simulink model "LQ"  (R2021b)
settings: Solver=VariableStepAuto  StartTime=0.0  StopTime=5  RelTol=1e-3
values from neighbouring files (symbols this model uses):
  a = 0.27    [CompareGazeboSimulink.m]    (also in RobotModel.m)
  b = 0.31    [CompareGazeboSimulink.m]    (also in RobotModel.m)
  desired_ang = 1    [RobotModel.m]
  desired_vel = 2    [RobotModel.m]
  distAng = 0    [RobotModel.m]
  distVel = 0    [RobotModel.m]
  fro = 0.02    [CompareGazeboSimulink.m]    (also in RobotModel.m)
  fsl = 0.8    [CompareGazeboSimulink.m]    (also in RobotModel.m)
  fsly = 0.8    [CompareGazeboSimulink.m]    (also in RobotModel.m)
  I = (1/12)*m*((2*t)^2 + 0.12^2) + 1.5    (= 2.384)    [CompareGazeboSimulink.m]    (also in RobotModel.m = 0.866666666667)
  k = 1    [RobotModel.m]
  ko = 0    [CompareGazeboSimulink.m]    (also in RobotModel.m = 0.25)
  kt = 0.58    [CompareGazeboSimulink.m]    (also in RobotModel.m)
  m = 51    [CompareGazeboSimulink.m]    (also in RobotModel.m = 50)
  mdy = 10    [CompareGazeboSimulink.m]    (also in RobotModel.m)
  mst = 10    [CompareGazeboSimulink.m]    (also in RobotModel.m)
  Q = [1 0    [RobotModel.m]
  r = 0.19    [CompareGazeboSimulink.m]    (also in RobotModel.m)
  R = [0.01 0    [RobotModel.m]
  T_vel_variance = 0.0005    [RobotModel.m]
  Th0 = 0    [CompareGazeboSimulink.m]    (also in RobotModel.m = 0.9714)
  Th_vel0 = 0    [CompareGazeboSimulink.m]    (also in RobotModel.m)
  Ts = 0.01    [CompareGazeboSimulink.m]    (also in RobotModel.m = 0.05)
  X0 = 0    [CompareGazeboSimulink.m]    (also in RobotModel.m)
  x_vel0 = 0    [CompareGazeboSimulink.m]    (also in RobotModel.m)
  x_vel_variance = 0.0005    [RobotModel.m]
  Y0 = 0    [CompareGazeboSimulink.m]    (also in RobotModel.m = 2.5)
libraries: mobileRoboticsLib x1

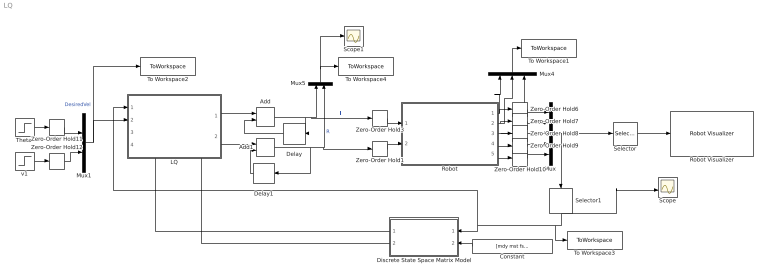
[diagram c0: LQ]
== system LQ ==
  Add : Sum
  Add1 : Sum
  Constant : Constant  Value=[mdy mst fsly r t a b m I Ts k]
  Delay : Delay  DelayLength=1
  Delay1 : Delay  DelayLength=1
  Discrete State Space Matrix Model : MATLAB Function  TreatAsAtomicUnit=on
  LQ : Subsystem
  Mux : Mux  Inputs=5
  Mux1 : Mux  Inputs=2
  Mux4 : Mux  Inputs=3
  Mux5 : Mux  Inputs=2
  Robot : Subsystem
  Robot Visualizer : mobileRoboticsLib/Environments/Robot Visualizer  robotRadius=0.3  showTrajectory=on  hasWaypoints=off  hasLidar=off  sensorOffset=[ 0, 0 ]  scanAngles=[ -pi/4, 0, pi/4 ]  hasObjDetector=off  objDetectorOffset=[ 0, 0 ]  objDetectorAngle=0  objDetectorFOV=pi/4  objDetectorMaxRange=5  objectColors=[ 1, 0, 0; 0, 1, 0; 0, 0, 1 ]  objectMarkers=s
  Scope : Scope  NumInputPorts=2
  Scope1 : Scope
  Selector : Selector  InputPortWidth=5  IndexOptions=Index vector (dialog)  Indices=[1 2 3]  OutputSizes=1
  Selector1 : Selector  InputPortWidth=5  IndexOptions=Index vector (dialog)  Indices=[4 5]  OutputSizes=1
  Theta' : Step  After=desired_ang  SampleTime=0
  To Workspace1 : ToWorkspace  VariableName=ActualPos  SaveFormat=Timeseries  SampleTime=-1
  To Workspace2 : ToWorkspace  VariableName=DesiredVel  SaveFormat=Timeseries  SampleTime=-1
  To Workspace3 : ToWorkspace  VariableName=ActualVel  SaveFormat=Timeseries  SampleTime=-1
  To Workspace4 : ToWorkspace  VariableName=Forces  SaveFormat=Timeseries  SampleTime=-1
  Zero-Order Hold{1,3,6..12} (9 alike) : ZeroOrderHold  SampleTime=Ts
  v1 : Step  After=desired_vel  SampleTime=0
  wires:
  Zero-Order Hold12/1 -> Mux1/2
  Zero-Order Hold11/1 -> Mux1/1
  Theta'/1 -> Zero-Order Hold11/1
  v1/1 -> Zero-Order Hold12/1
  Mux4/1 -> To Workspace1/1
  Selector1/1 -> Scope/2, To Workspace3/1, LQ/1(Actual State), Discrete State Space Matrix Model/1(State)
  Discrete State Space Matrix Model/1(A) -> LQ/3(A)
  Robot/5(v) -> Zero-Order Hold10/1
  Robot/4(Theta') -> Zero-Order Hold9/1
  Selector/1 -> Robot Visualizer/1
  Mux1/1 -> To Workspace2/1, LQ/2(Desired State)  "DesiredVel"
  Zero-Order Hold7/1 -> Mux/2
  Robot/2(Y) -> Mux4/2, Zero-Order Hold7/1
  Delay/1 -> Add/2
  Zero-Order Hold10/1 -> Mux/5
  Robot/1(X) -> Mux4/1, Zero-Order Hold6/1
  Zero-Order Hold1/1 -> Robot/2(Right Force)
  Zero-Order Hold6/1 -> Mux/1
  Zero-Order Hold8/1 -> Mux/3
  Delay1/1 -> Add1/2
  Add/1 -> Mux5/1, Zero-Order Hold3/1, Delay/1  "L"
  Zero-Order Hold9/1 -> Mux/4
  Discrete State Space Matrix Model/2(B) -> LQ/4(B)
  Robot/3(Theta) -> Mux4/3, Zero-Order Hold8/1
  LQ/2(Right Force) -> Add1/1
  Zero-Order Hold3/1 -> Robot/1(Left Force)
  LQ/1(" Left Force") -> Add/1
  Mux/1 -> Selector/1, Selector1/1
  Constant/1 -> Discrete State Space Matrix Model/2(param)
  Add1/1 -> Zero-Order Hold1/1, Mux5/2, Delay1/1  "R"
  Mux5/1 -> To Workspace4/1, Scope1/1

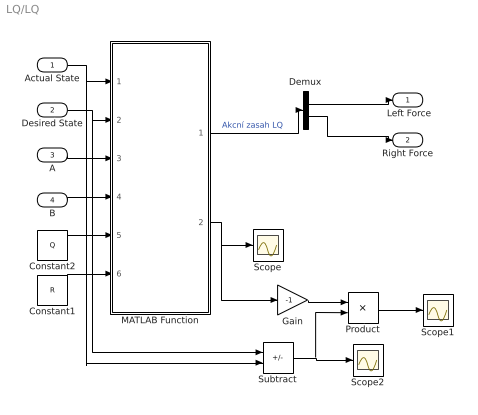
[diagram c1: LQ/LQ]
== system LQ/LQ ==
  Actual State : Inport
  Desired State : Inport  Port=2
  A : Inport  Port=3
  B : Inport  Port=4
  Constant1 : Constant  Value=R
  Constant2 : Constant  Value=Q
  Demux : Demux  Outputs=2
  Gain : Gain  Gain=-1
  MATLAB Function : MATLAB Function  TreatAsAtomicUnit=on
  Product : Product  Multiplication=Matrix(*)
  Scope : Scope
  Scope1 : Scope
  Scope2 : Scope
  Subtract : Sum  Inputs=+-
  " Left Force" : Outport
  Right Force : Outport  Port=2
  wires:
  MATLAB Function/1(u) -> Demux/1  "Akcní zasah LQ"
  Actual State/1 -> Subtract/2, MATLAB Function/1(ActualState)
  Desired State/1 -> Subtract/1, MATLAB Function/2(DesiredState)
  A/1 -> MATLAB Function/3(A)
  B/1 -> MATLAB Function/4(B)
  Constant2/1 -> MATLAB Function/5(Q)
  Constant1/1 -> MATLAB Function/6(R)
  MATLAB Function/2(K) -> Gain/1, Scope/1
  Subtract/1 -> Scope2/1, Product/2
  Gain/1 -> Product/1
  Product/1 -> Scope1/1
  Demux/1 -> " Left Force"/1
  Demux/2 -> Right Force/1

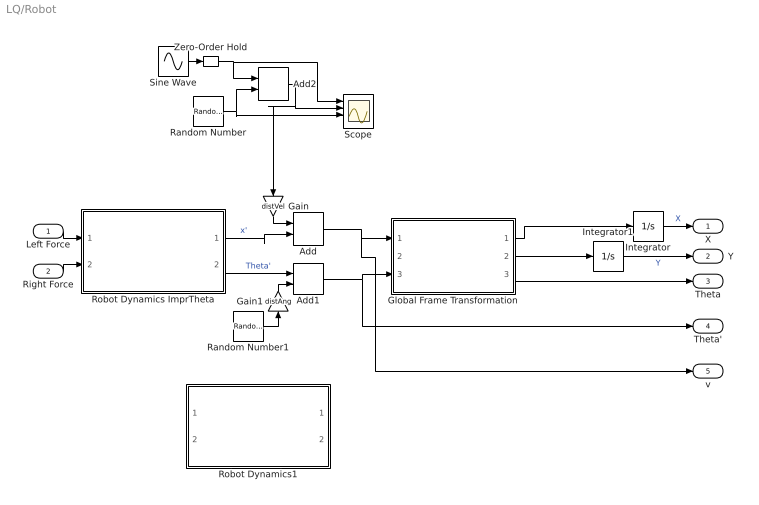
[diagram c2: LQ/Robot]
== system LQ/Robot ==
  Left Force : Inport
  Right Force : Inport  Port=2
  Add : Sum
  Add1 : Sum
  Add2 : Sum
  Gain : Gain  Gain=distVel
  Gain1 : Gain  Gain=distAng
  Global Frame Transformation : Subsystem
  Integrator : Integrator  InitialCondition=X0
  Integrator1 : Integrator  InitialCondition=Y0
  Random Number : RandomNumber  Variance=x_vel_variance  SampleTime=0.2
  Random Number1 : RandomNumber  Variance=T_vel_variance  SampleTime=0.2
  Robot Dynamics ImprTheta : Subsystem
  Robot Dynamics1 : Subsystem  Commented=on
  Scope : Scope  NumInputPorts=4
  Sine Wave : Sin  Amplitude=0.1*desired_vel  Frequency=0.2  SampleTime=0
  Zero-Order Hold : ZeroOrderHold  SampleTime=0.25
  X : Outport
  Y : Outport  Port=2
  Theta : Outport  Port=3
  Theta' : Outport  Port=4
  v : Outport  Port=5
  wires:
  Right Force/1 -> Robot Dynamics ImprTheta/2(Right Force)
  Global Frame Transformation/1(X') -> Integrator/1
  Integrator/1 -> X/1  "X"
  Left Force/1 -> Robot Dynamics ImprTheta/1(Left Force)
  Global Frame Transformation/2(Y') -> Integrator1/1
  Global Frame Transformation/3(Theta) -> Theta/1
  Integrator1/1 -> Y/1  "Y"
  Robot Dynamics ImprTheta/1(x') -> Add/2  "x'"
  Add/1 -> v/1, Global Frame Transformation/1(x')
  Robot Dynamics ImprTheta/2(Theta') -> Add1/1  "Theta'"
  Add1/1 -> Theta'/1, Global Frame Transformation/3(Theta')
  Random Number1/1 -> Gain1/1
  Random Number/1 -> Add2/2, Scope/3
  Add2/1 -> Gain/1, Scope/2
  Sine Wave/1 -> Zero-Order Hold/1
  Zero-Order Hold/1 -> Scope/1, Add2/1
  Gain/1 -> Add/1
  Gain1/1 -> Add1/2

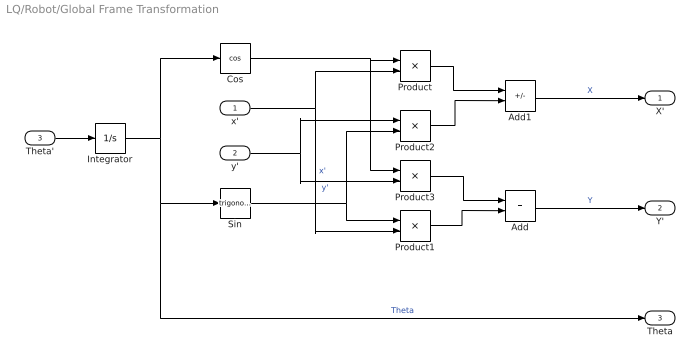
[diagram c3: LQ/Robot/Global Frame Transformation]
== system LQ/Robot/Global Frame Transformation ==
  x' : Inport
  y' : Inport  Port=2
  Theta' : Inport  Port=3
  Add : Sum
  Add1 : Sum  Inputs=+-
  Cos : Trigonometry  Operator=cos
  Integrator : Integrator  InitialCondition=Th0
  Product{,1..3} (4 alike) : Product
  Sin : Trigonometry
  X' : Outport
  Y' : Outport  Port=2
  Theta : Outport  Port=3
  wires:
  Add/1 -> Y'/1  "Y"
  Integrator/1 -> Theta/1, Sin/1, Cos/1  "Theta"
  Product1/1 -> Add/2
  x'/1 -> Product/2, Product1/2  "x'"
  Sin/1 -> Product1/1, Product2/2
  Product2/1 -> Add1/2
  Product3/1 -> Add/1
  Product/1 -> Add1/1
  Cos/1 -> Product/1, Product3/1
  y'/1 -> Product3/2, Product2/1  "y'"
  Add1/1 -> X'/1  "X"
  Theta'/1 -> Integrator/1

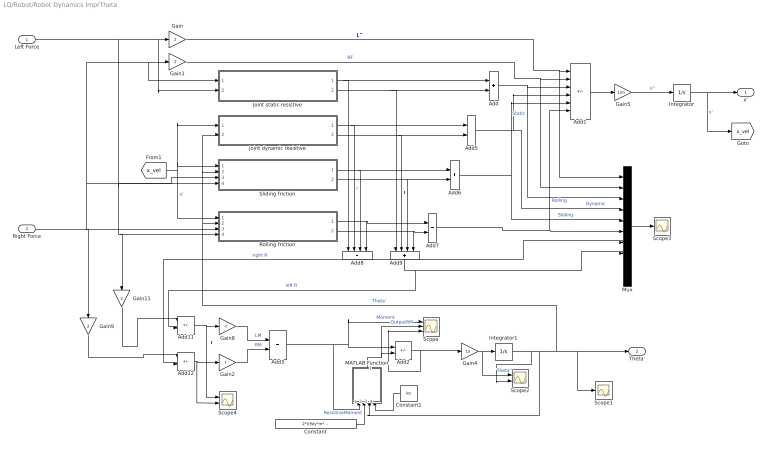
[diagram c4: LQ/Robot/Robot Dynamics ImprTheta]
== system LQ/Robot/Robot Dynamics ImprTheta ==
  Left Force : Inport
  Right Force : Inport  Port=2
  Add{,3,5..7} (5 alike) : Sum
  Add1 : Sum  Inputs=++----
  Add11 : Sum  Inputs=+-
  Add12 : Sum  Inputs=+-
  Add2 : Sum  Inputs=+-
  Add8 : Sum  Inputs=++++
  Add9 : Sum  Inputs=++++
  Constant : Constant  Value=2*((fsly*m*9.81)/(a+b))*a*b*kt
  Constant1 : Constant  Value=ko
  Gain{,1,9,11} (4 alike) : Gain  Gain=2
  Gain2 : Gain  Gain=t
  Gain4 : Gain  Gain=1/I
  Gain5 : Gain  Gain=1/m
  Gain8 : Gain  Gain=-t
  Integrator : Integrator  InitialCondition=x_vel0
  Integrator1 : Integrator  InitialCondition=Th_vel0
  Joint dynamic resistive : Subsystem
  Joint static resistive : Subsystem
  MATLAB Function : MATLAB Function  TreatAsAtomicUnit=on
  Mux : Mux  Inputs=10
  Rolling friction : Subsystem
  Scope : Scope  NumInputPorts=3
  Scope1 : Scope
  Scope2 : Scope  NumInputPorts=2
  Scope3 : Scope
  Scope4 : Scope  NumInputPorts=2
  Sliding friction : Subsystem
  x' : Outport
  Theta' : Outport  Port=2
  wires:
  Gain4/1 -> Scope2/1, Integrator1/1  "Theta''"
  Integrator1/1 -> Scope2/2, Sliding friction/2(Theta'), Joint dynamic resistive/2(Theta'), Rolling friction/2(Theta'), Scope1/1, Theta'/1, MATLAB Function/3(Omega)  "Theta'"
  Gain1/1 -> Mux/2, Add1/2  "RF"
  Add1/1 -> Gain5/1
  Gain5/1 -> Integrator/1  "x''"
  Integrator/1 -> x'/1, [x_vel]  "x'"
  [x_vel] -> Joint dynamic resistive/1("Local Long Velocity "), Sliding friction/1(Local longitudal velocity), Rolling friction/1(Local longitudal velocity)  "x'"
  Joint static resistive/2(Static Resistive Force Left) -> Add9/1, Add/2
  Joint dynamic resistive/1(Dynamic Resistive Force Right) -> Add8/2, Add5/1  "r"
  Joint dynamic resistive/2(Dynamic Resistive Force Left) -> Add9/2, Add5/2  "l"
  Sliding friction/1(Friction Right Force) -> Add8/3, Add6/1
  Sliding friction/2(Friction Left Force) -> Add9/3, Add6/2
  Rolling friction/1(Friction Right Force) -> Add8/4, Add7/1
  Rolling friction/2(Friction Left Force) -> Add9/4, Add7/2
  Add/1 -> Add1/3, Mux/3  "Static"
  Add6/1 -> Add1/5, Mux/5  "Sliding"
  Add7/1 -> Mux/6, Add1/6  "Rolling"
  Add5/1 -> Mux/4, Add1/4  "Dynamic"
  Add9/1 -> Add11/2, Mux/8  "left R"
  Add8/1 -> Add12/2, Mux/7  "right R"
  Mux/1 -> Scope3/1
  Add11/1 -> Scope4/1, Gain8/1  "LL"
  Add12/1 -> Scope4/2, Gain2/1
  Gain9/1 -> Add12/1
  Gain11/1 -> Add11/1
  Gain8/1 -> Add3/1  "LM"
  Gain2/1 -> Add3/2  "RM"
  Gain/1 -> Mux/1, Add1/1  "LF"
  Joint static resistive/1(Static Resistive Force Right) -> Add8/1, Add/1
  Add2/1 -> Scope/3, Gain4/1
  Add3/1 -> Scope/1, Add2/1, MATLAB Function/1(Moment)  "Moment"
  MATLAB Function/1(y) -> Scope/2, Add2/2  "OutputRM"
  Constant/1 -> MATLAB Function/2(ResistiveMoment)  "ResistiveMoment"
  Left Force/1 -> Gain11/1, Rolling friction/4(Fl), Sliding friction/4(Fl), Joint static resistive/2("Fl "), Gain/1
  Right Force/1 -> Gain9/1, Rolling friction/3(Fr), Sliding friction/3(Fr), Joint static resistive/1(Fr), Gain1/1
  Constant1/1 -> MATLAB Function/4(ko)

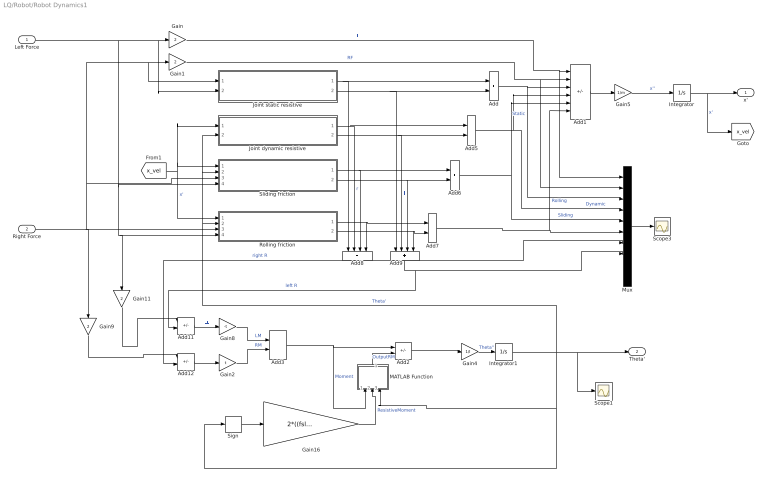
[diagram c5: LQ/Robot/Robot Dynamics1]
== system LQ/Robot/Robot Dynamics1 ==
  Left Force : Inport
  Right Force : Inport  Port=2
  Add{,3,5..7} (5 alike) : Sum
  Add1 : Sum  Inputs=++----
  Add11 : Sum  Inputs=+-
  Add12 : Sum  Inputs=+-
  Add2 : Sum  Inputs=+-
  Add8 : Sum  Inputs=++++
  Add9 : Sum  Inputs=++++
  Gain{,1,9,11} (4 alike) : Gain  Gain=2
  Gain16 : Gain  Gain=2*((fsly*m*9.81)/(a+b))*a*b
  Gain2 : Gain  Gain=t
  Gain4 : Gain  Gain=1/I
  Gain5 : Gain  Gain=1/m
  Gain8 : Gain  Gain=-t
  Integrator : Integrator  InitialCondition=x_vel0
  Integrator1 : Integrator  InitialCondition=Th_vel0
  Joint dynamic resistive : Subsystem
  Joint static resistive : Subsystem
  MATLAB Function : MATLAB Function  TreatAsAtomicUnit=on
  Mux : Mux  Inputs=10
  Rolling friction : Subsystem
  Scope1 : Scope
  Scope3 : Scope
  Sign : Signum
  Sliding friction : Subsystem
  x' : Outport
  Theta' : Outport  Port=2
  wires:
  Right Force/1 -> Rolling friction/3(Fr), Sliding friction/3(Fr), Joint static resistive/1(Fr), Gain1/1, Gain9/1
  Gain4/1 -> Integrator1/1  "Theta''"
  Integrator1/1 -> Sliding friction/2(Theta'), Joint dynamic resistive/2(Theta'), Rolling friction/2(Theta'), MATLAB Function/3(Omega), Sign/1, Scope1/1, Theta'/1  "Theta'"
  Left Force/1 -> Rolling friction/4(Fl), Gain11/1, Sliding friction/4(Fl), Joint static resistive/2("Fl "), Gain/1
  Gain1/1 -> Mux/2, Add1/2  "RF"
  Add1/1 -> Gain5/1
  Gain5/1 -> Integrator/1  "x''"
  Integrator/1 -> x'/1, [x_vel]  "x'"
  [x_vel] -> Joint dynamic resistive/1("Local Long Velocity "), Sliding friction/1(Local longitudal velocity), Rolling friction/1(Local longitudal velocity)  "x'"
  Joint static resistive/2(Static Resistive Force Left) -> Add9/1, Add/2
  Joint dynamic resistive/1(Dynamic Resistive Force Right) -> Add8/2, Add5/1  "r"
  Joint dynamic resistive/2(Dynamic Resistive Force Left) -> Add9/2, Add5/2  "l"
  Sliding friction/1(Friction Right Force) -> Add8/3, Add6/1
  Sliding friction/2(Friction Left Force) -> Add9/3, Add6/2
  Rolling friction/1(Friction Right Force) -> Add8/4, Add7/1
  Rolling friction/2(Friction Left Force) -> Add9/4, Add7/2
  Add/1 -> Add1/3, Mux/3  "Static"
  Add6/1 -> Add1/5, Mux/5  "Sliding"
  Add7/1 -> Mux/6, Add1/6  "Rolling"
  Add5/1 -> Mux/4, Add1/4  "Dynamic"
  Add9/1 -> Add11/2, Mux/8  "left R"
  Add8/1 -> Add12/2, Mux/7  "right R"
  Mux/1 -> Scope3/1
  Add11/1 -> Gain8/1  "LL"
  Add12/1 -> Gain2/1
  Gain9/1 -> Add12/1
  Gain11/1 -> Add11/1
  Gain8/1 -> Add3/1  "LM"
  Gain2/1 -> Add3/2  "RM"
  Gain/1 -> Mux/1, Add1/1  "LF"
  Joint static resistive/1(Static Resistive Force Right) -> Add8/1, Add/1
  Sign/1 -> Gain16/1
  Add2/1 -> Gain4/1
  Add3/1 -> Add2/1, MATLAB Function/1(Moment)  "Moment"
  MATLAB Function/1(y) -> Add2/2  "OutputRM"
  Gain16/1 -> MATLAB Function/2(ResistiveMoment)  "ResistiveMoment"

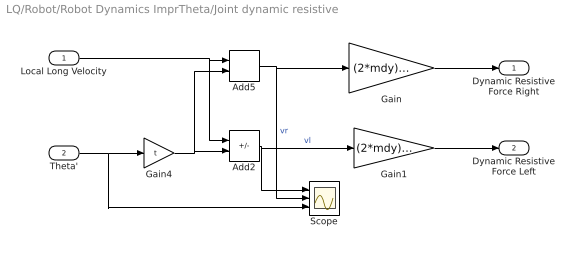
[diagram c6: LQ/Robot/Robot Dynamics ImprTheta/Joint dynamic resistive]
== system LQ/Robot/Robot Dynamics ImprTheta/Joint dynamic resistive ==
  "Local Long Velocity " : Inport
  Theta' : Inport  Port=2
  Add2 : Sum  Inputs=+-
  Add5 : Sum
  Gain : Gain  Gain=(2*mdy)/(r*r)
  Gain1 : Gain  Gain=(2*mdy)/(r*r)
  Gain4 : Gain  Gain=t
  Scope : Scope  NumInputPorts=3
  Dynamic Resistive Force Right : Outport
  Dynamic Resistive Force Left : Outport  Port=2
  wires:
  Gain/1 -> Dynamic Resistive Force Right/1
  Gain1/1 -> Dynamic Resistive Force Left/1
  Gain4/1 -> Add5/2, Add2/2
  Theta'/1 -> Scope/3, Gain4/1
  Add5/1 -> Scope/2, Gain/1  "vr"
  Add2/1 -> Scope/1, Gain1/1  "vl"
  "Local Long Velocity "/1 -> Add2/1, Add5/1

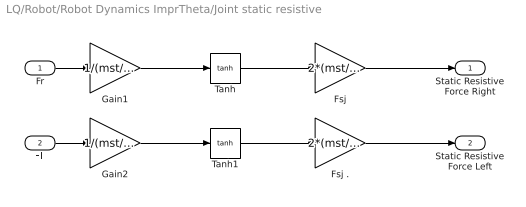
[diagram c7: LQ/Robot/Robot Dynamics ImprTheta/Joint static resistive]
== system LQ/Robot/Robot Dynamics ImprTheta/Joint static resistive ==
  Fr : Inport
  "Fl " : Inport  Port=2
  Fsj : Gain  Gain=2*(mst/r)
  Fsj . : Gain  Gain=2*(mst/r)
  Gain1 : Gain  Gain=1/(mst/r)
  Gain2 : Gain  Gain=1/(mst/r)
  Tanh : Trigonometry  Operator=tanh
  Tanh1 : Trigonometry  Operator=tanh
  Static Resistive Force Right : Outport
  Static Resistive Force Left : Outport  Port=2
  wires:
  Fr/1 -> Gain1/1
  "Fl "/1 -> Gain2/1
  Tanh/1 -> Fsj/1
  Tanh1/1 -> Fsj ./1
  Gain1/1 -> Tanh/1
  Gain2/1 -> Tanh1/1
  Fsj/1 -> Static Resistive Force Right/1
  Fsj ./1 -> Static Resistive Force Left/1

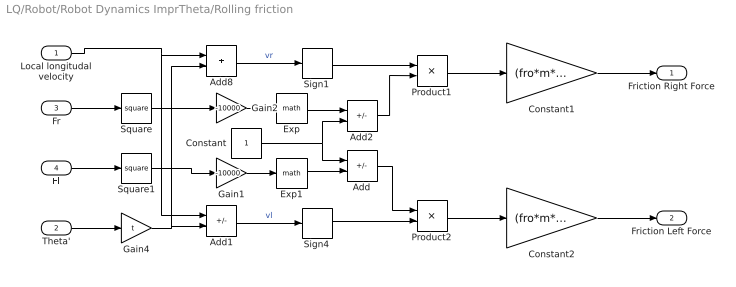
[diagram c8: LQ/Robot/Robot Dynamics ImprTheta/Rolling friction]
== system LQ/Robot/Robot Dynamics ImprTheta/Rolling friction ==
  Local longitudal velocity : Inport
  Theta' : Inport  Port=2
  Fr : Inport  Port=3
  Fl : Inport  Port=4
  Add : Sum  Inputs=+-
  Add1 : Sum  Inputs=+-
  Add2 : Sum  Inputs=-+
  Add8 : Sum
  Constant : Constant
  Constant1 : Gain  Gain=(fro*m*9.81)/2
  Constant2 : Gain  Gain=(fro*m*9.81)/2
  Exp : Math
  Exp1 : Math
  Gain1 : Gain  Gain=-10000
  Gain2 : Gain  Gain=-10000
  Gain4 : Gain  Gain=t
  Product1 : Product
  Product2 : Product
  Sign1 : Signum
  Sign4 : Signum
  Square : Math  Operator=square
  Square1 : Math  Operator=square
  Friction Right Force : Outport
  Friction Left Force : Outport  Port=2
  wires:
  Sign1/1 -> Product1/1
  Sign4/1 -> Product2/2
  Add8/1 -> Sign1/1  "vr"
  Fl/1 -> Square1/1
  Fr/1 -> Square/1
  Square1/1 -> Gain1/1
  Gain4/1 -> Add1/2, Add8/2
  Theta'/1 -> Gain4/1
  Add1/1 -> Sign4/1  "vl"
  Square/1 -> Gain2/1
  Gain2/1 -> Exp/1
  Gain1/1 -> Exp1/1
  Add2/1 -> Product1/2
  Add/1 -> Product2/1
  Exp1/1 -> Add/2
  Exp/1 -> Add2/1
  Constant/1 -> Add2/2, Add/1
  Local longitudal velocity/1 -> Add1/1, Add8/1
  Product1/1 -> Constant1/1
  Product2/1 -> Constant2/1
  Constant2/1 -> Friction Left Force/1
  Constant1/1 -> Friction Right Force/1

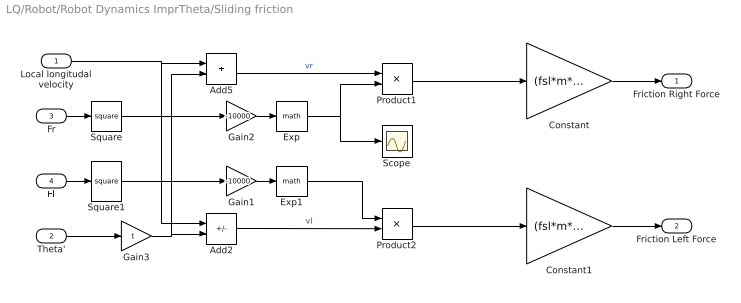
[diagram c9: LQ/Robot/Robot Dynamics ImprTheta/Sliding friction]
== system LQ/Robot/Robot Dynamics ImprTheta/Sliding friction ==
  Local longitudal velocity : Inport
  Theta' : Inport  Port=2
  Fr : Inport  Port=3
  Fl : Inport  Port=4
  Add2 : Sum  Inputs=+-
  Add5 : Sum
  Constant : Gain  Gain=(fsl*m*9.81)/2
  Constant1 : Gain  Gain=(fsl*m*9.81)/2
  Exp : Math
  Exp1 : Math
  Gain1 : Gain  Gain=-10000
  Gain2 : Gain  Gain=-10000
  Gain3 : Gain  Gain=t
  Product1 : Product
  Product2 : Product
  Scope : Scope
  Square : Math  Operator=square
  Square1 : Math  Operator=square
  Friction Right Force : Outport
  Friction Left Force : Outport  Port=2
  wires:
  Theta'/1 -> Gain3/1
  Gain3/1 -> Add2/2, Add5/2
  Add5/1 -> Product1/1  "vr"
  Add2/1 -> Product2/2  "vl"
  Exp/1 -> Scope/1, Product1/2
  Gain1/1 -> Exp1/1
  Gain2/1 -> Exp/1
  Fr/1 -> Square/1
  Fl/1 -> Square1/1
  Square/1 -> Gain2/1
  Square1/1 -> Gain1/1
  Product1/1 -> Constant/1
  Product2/1 -> Constant1/1
  Exp1/1 -> Product2/1
  Local longitudal velocity/1 -> Add2/1, Add5/1
  Constant/1 -> Friction Right Force/1
  Constant1/1 -> Friction Left Force/1

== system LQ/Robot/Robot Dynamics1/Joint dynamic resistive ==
  "Local Long Velocity " : Inport
  Theta' : Inport  Port=2
  Add2 : Sum  Inputs=+-
  Add5 : Sum
  Gain : Gain  Gain=(2*mdy)/(r*r)
  Gain1 : Gain  Gain=(2*mdy)/(r*r)
  Gain4 : Gain  Gain=t
  Scope : Scope  NumInputPorts=3
  Dynamic Resistive Force Right : Outport
  Dynamic Resistive Force Left : Outport  Port=2
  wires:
  Gain/1 -> Dynamic Resistive Force Right/1
  Gain1/1 -> Dynamic Resistive Force Left/1
  Gain4/1 -> Add5/2, Add2/2
  Theta'/1 -> Scope/3, Gain4/1
  Add5/1 -> Scope/2, Gain/1  "vr"
  Add2/1 -> Scope/1, Gain1/1  "vl"
  "Local Long Velocity "/1 -> Add2/1, Add5/1

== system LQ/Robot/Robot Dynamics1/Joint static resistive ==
  Fr : Inport
  "Fl " : Inport  Port=2
  Fsj : Gain  Gain=2*(mst/r)
  Fsj . : Gain  Gain=2*(mst/r)
  Gain1 : Gain  Gain=1/(mst/r)
  Gain2 : Gain  Gain=1/(mst/r)
  Tanh : Trigonometry  Operator=tanh
  Tanh1 : Trigonometry  Operator=tanh
  Static Resistive Force Right : Outport
  Static Resistive Force Left : Outport  Port=2
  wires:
  Fr/1 -> Gain1/1
  "Fl "/1 -> Gain2/1
  Tanh/1 -> Fsj/1
  Tanh1/1 -> Fsj ./1
  Gain1/1 -> Tanh/1
  Gain2/1 -> Tanh1/1
  Fsj/1 -> Static Resistive Force Right/1
  Fsj ./1 -> Static Resistive Force Left/1

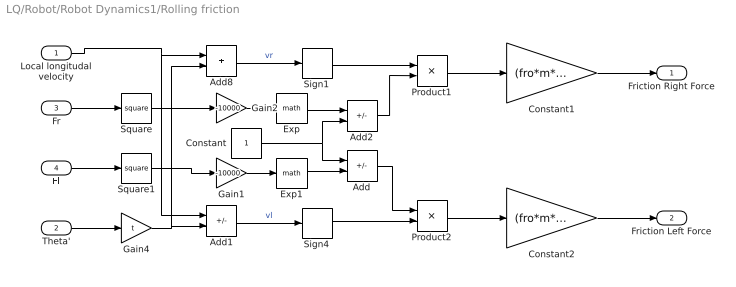
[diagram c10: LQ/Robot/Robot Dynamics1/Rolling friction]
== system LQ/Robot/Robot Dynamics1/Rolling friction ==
  Local longitudal velocity : Inport
  Theta' : Inport  Port=2
  Fr : Inport  Port=3
  Fl : Inport  Port=4
  Add : Sum  Inputs=+-
  Add1 : Sum  Inputs=+-
  Add2 : Sum  Inputs=-+
  Add8 : Sum
  Constant : Constant
  Constant1 : Gain  Gain=(fro*m*9.81)/2
  Constant2 : Gain  Gain=(fro*m*9.81)/2
  Exp : Math
  Exp1 : Math
  Gain1 : Gain  Gain=-10000
  Gain2 : Gain  Gain=-10000
  Gain4 : Gain  Gain=t
  Product1 : Product
  Product2 : Product
  Sign1 : Signum
  Sign4 : Signum
  Square : Math  Operator=square
  Square1 : Math  Operator=square
  Friction Right Force : Outport
  Friction Left Force : Outport  Port=2
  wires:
  Sign1/1 -> Product1/1
  Sign4/1 -> Product2/2
  Add8/1 -> Sign1/1  "vr"
  Fl/1 -> Square1/1
  Fr/1 -> Square/1
  Square1/1 -> Gain1/1
  Gain4/1 -> Add1/2, Add8/2
  Theta'/1 -> Gain4/1
  Add1/1 -> Sign4/1  "vl"
  Square/1 -> Gain2/1
  Gain2/1 -> Exp/1
  Gain1/1 -> Exp1/1
  Add2/1 -> Product1/2
  Add/1 -> Product2/1
  Exp1/1 -> Add/2
  Exp/1 -> Add2/1
  Constant/1 -> Add2/2, Add/1
  Local longitudal velocity/1 -> Add1/1, Add8/1
  Product1/1 -> Constant1/1
  Product2/1 -> Constant2/1
  Constant2/1 -> Friction Left Force/1
  Constant1/1 -> Friction Right Force/1

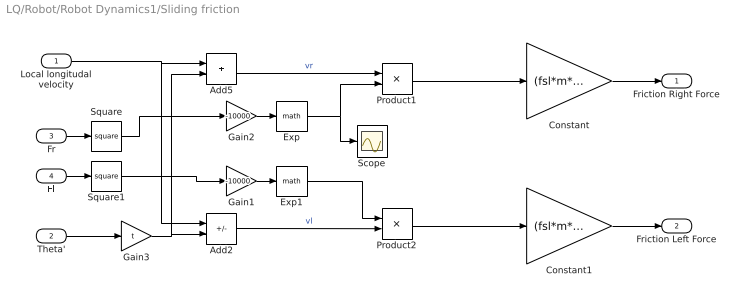
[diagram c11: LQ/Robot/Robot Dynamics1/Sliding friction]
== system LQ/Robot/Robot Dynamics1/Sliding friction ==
  Local longitudal velocity : Inport
  Theta' : Inport  Port=2
  Fr : Inport  Port=3
  Fl : Inport  Port=4
  Add2 : Sum  Inputs=+-
  Add5 : Sum
  Constant : Gain  Gain=(fsl*m*9.81)/2
  Constant1 : Gain  Gain=(fsl*m*9.81)/2
  Exp : Math
  Exp1 : Math
  Gain1 : Gain  Gain=-10000
  Gain2 : Gain  Gain=-10000
  Gain3 : Gain  Gain=t
  Product1 : Product
  Product2 : Product
  Scope : Scope
  Square : Math  Operator=square
  Square1 : Math  Operator=square
  Friction Right Force : Outport
  Friction Left Force : Outport  Port=2
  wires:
  Theta'/1 -> Gain3/1
  Gain3/1 -> Add2/2, Add5/2
  Add5/1 -> Product1/1  "vr"
  Add2/1 -> Product2/2  "vl"
  Exp/1 -> Scope/1, Product1/2
  Gain1/1 -> Exp1/1
  Gain2/1 -> Exp/1
  Fr/1 -> Square/1
  Fl/1 -> Square1/1
  Square/1 -> Gain2/1
  Square1/1 -> Gain1/1
  Product1/1 -> Constant/1
  Product2/1 -> Constant1/1
  Exp1/1 -> Product2/1
  Local longitudal velocity/1 -> Add2/1, Add5/1
  Constant/1 -> Friction Right Force/1
  Constant1/1 -> Friction Left Force/1

== matlab function LQ/Discrete State Space
Matrix Model ==
function [A, B] = fcn(State, param)  
    mdy = param(1);
    mst = param(2);
    fsly = param(3);
    r = param(4);
    t = param(5);
    a = param(6);
    b = param(7);
    m = param(8);
    I = param(9);
    Ts = param(10);
    k = param(11);
    
    O = State(1);
    
    A = eye(2) + [(-4*(mdy/(r*r))*t*t -2*(fsly*m*9.81/(a+b))*a*b)/I 0 ;
                  0 -4*(mdy/(r*r))/m]*Ts;

    % -2*(fsly*m*9.81/(a+b))*a*b*(2/3.14159)*(2/(1+2*2*O*O))
    B = Ts*[-2*t/I 2*t/I; 2/m 2/m];
end

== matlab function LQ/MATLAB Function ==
function [u, K] = lq(ActualState, DesiredState, A, B, Q, R)                                                     

K_old = [ 0 0;
          0 0];
K     = [1 1;
         1 1];

P = [1 0; 0 1];
i = 0;
while (K ~= K_old)
    i = i + 1;
    K_old = K;
    %P = Q + K'*R*K + (A - B*K)'*P*(A - B*K);
    P = A'*P*A - (A'*P*B)*(R+B'*P*B)^(-1)*(B'*P*A) + Q;
    K = (R + B'*P*B)^(-1)*B'*P*A;

    if (i > 500)
        break
    end
end

u = -K*(DesiredState - ActualState);
end

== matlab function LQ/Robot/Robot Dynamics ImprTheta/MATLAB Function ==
function y = fcn(Moment, ResistiveMoment, Omega, ko)
    y = Omega*ResistiveMoment;

%     if(abs(Moment) < abs(ResistiveMoment))
%         y = Moment;
%     else
%         y = (ko*Omega + sign(Omega))*ResistiveMoment;
%     end



end

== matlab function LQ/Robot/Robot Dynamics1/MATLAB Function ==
function y = fcn(Moment, ResistiveMoment, Omega)
    y = ResistiveMoment;
    
    if(Omega ~= 0)
        if(abs(Moment) < abs(ResistiveMoment))
            y = sign(Omega)*abs(Moment);
        else
            y = ResistiveMoment;
        end
    else
        y = 0;


end
